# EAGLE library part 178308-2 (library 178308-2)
20 Positions Header Connector 0.150" (3.81mm) Through Hole, Right Angle Gold Source: Datasheet
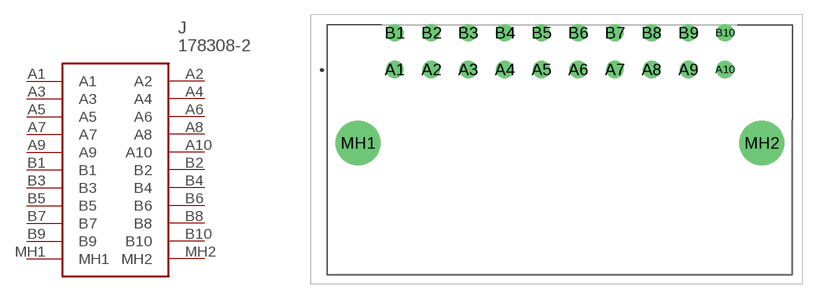
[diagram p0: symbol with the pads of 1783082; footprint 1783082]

Designator prefix J

## 178308-2 (Description: 20 Positions Header Connector 0.150" (3.81mm) Through Hole, Right Angle Gold; Height: 14mm; Manufacturer_Name: TE Connectivity; Manufacturer_Part_Number: 178308-2; Mouser_Part_Number: 571-1783082; Mouser_Price-Stock: https://www.mouser.com/Search/Refine.aspx?Keyword=571-1783082)  [1783082]
A1  A1
A2  A2
A3  A3
A4  A4
A5  A5
A6  A6
A7  A7
A8  A8
A9  A9
A10  A10
B1  B1
B2  B2
B3  B3
B4  B4
B5  B5
B6  B6
B7  B7
B8  B8
B9  B9
B10  B10
MH1  MH1
MH2  MH2

## Footprint 1783082 (pad centres in mm)
178308-2
drill 1.2 pad 1.8: A1 -16.817,8.285; A2 -13.007,8.285; A3 -9.197,8.285; A4 -5.387,8.285; A5 -1.577,8.285; A6 2.233,8.285; A7 6.043,8.285; A8 9.853,8.285; A9 13.663,8.285; A10 17.473,8.285; B1 -16.817,12.095; B2 -13.007,12.095; B3 -9.197,12.095; B4 -5.387,12.095; B5 -1.577,12.095; B6 2.233,12.095; B7 6.043,12.095; B8 9.853,12.095; B9 13.663,12.095; B10 17.473,12.095
drill 3.1 pad 4.65: MH1 -20.627,0.665; MH2 21.283,0.665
